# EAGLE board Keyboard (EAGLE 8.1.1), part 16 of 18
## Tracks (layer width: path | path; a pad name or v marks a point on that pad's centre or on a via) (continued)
S$16561 (continued)
  Bottom 0: 240.03,79.83 248.76,71.09
S$16562
  Bottom 0: 248.76,71.09 248.82,71.05
S$16563
  Bottom 0: 248.82,71.05 248.88,71.01
S$16564
  Bottom 0: 248.88,71.01 248.94,70.98
S$16565
  Bottom 0: 248.94,70.98 249.01,70.97
S$16566
  Bottom 0: 249.01,70.97 249.08,70.97
S$16567
  Bottom 0: 249.08,70.97 251.03,70.97
S$16568
  Bottom 0: 251.03,70.97 255.22,66.77
S$16569
  Bottom 0: 255.22,66.77 255.27,66.73
S$16570
  Bottom 0: 255.27,66.73 255.33,66.69
S$16571
  Bottom 0: 255.33,66.69 255.39,66.66
S$16572
  Bottom 0: 255.39,66.66 255.46,66.65
S$16573
  Bottom 0: 255.46,66.65 255.53,66.64
S$16574
  Bottom 0: 255.53,66.64 259.04,66.64
S$16575
  Bottom 0: 259.04,66.64 259.11,66.65
S$16576
  Bottom 0: 259.11,66.65 259.17,66.66
S$16577
  Bottom 0: 259.17,66.66 259.23,66.69
S$16578
  Bottom 0: 259.23,66.69 259.29,66.72
S$16579
  Bottom 0: 259.29,66.72 259.35,66.77
S$16580
  Bottom 0: 259.35,66.77 259.7,67.11
S$16581
  Bottom 0: 259.7,67.11 260.5,67.11
S$16582
  Bottom 0: 260.5,67.11 260.44,67.06
S$16583
  Bottom 0: 260.44,67.06 260.27,66.81
S$16584
  Bottom 0: 260.27,66.81 260.18,66.53
S$16585
  Bottom 0: 260.18,66.53 260.18,66.22
S$16586
  Bottom 0: 260.18,66.22 260.27,65.93
S$16587
  Bottom 0: 260.27,65.93 260.44,65.68
S$16588
  Bottom 0: 260.44,65.68 260.68,65.49
S$16589
  Bottom 0: 260.68,65.49 260.96,65.38
S$16590
  Bottom 0: 260.96,65.38 261.26,65.36
S$16591
  Bottom 0: 261.26,65.36 261.56,65.43
S$16592
  Bottom 0: 261.56,65.43 261.82,65.58
S$16593
  Bottom 0: 261.82,65.58 262.02,65.8
S$16594
  Bottom 0: 262.02,65.8 262.15,66.07
S$16595
  Bottom 0: 262.15,66.07 262.2,66.37
S$16596
  Bottom 0: 262.2,66.37 262.15,66.67
S$16597
  Bottom 0: 262.15,66.67 262.02,66.94
S$16598
  Bottom 0: 262.02,66.94 261.87,67.11
S$16599
  Bottom 0: 261.87,67.11 264.83,67.11
S$16600
  Bottom 0: 264.83,67.11 265.05,66.9
S$16601
  Bottom 0: 265.05,66.9 265.1,66.86
S$16602
  Bottom 0: 265.1,66.86 265.16,66.81
S$16603
  Bottom 0: 265.16,66.81 265.22,66.79
S$16604
  Bottom 0: 265.22,66.79 265.29,66.77
S$16605
  Bottom 0: 265.29,66.77 265.36,66.77
S$16606
  Bottom 0: 265.36,66.77 268.52,66.77
S$16607
  Bottom 0: 268.52,66.77 268.22,66.61
S$16608
  Bottom 0: 268.22,66.61 267.88,66.32
S$16609
  Bottom 0: 267.88,66.32 267.59,65.98
S$16610
  Bottom 0: 267.59,65.98 267.38,65.58
S$16611
  Bottom 0: 267.38,65.58 267.25,65.15
S$16612
  Bottom 0: 267.25,65.15 267.2,64.71
S$16613
  Bottom 0: 267.2,64.71 267.25,64.26
S$16614
  Bottom 0: 267.25,64.26 267.38,63.83
S$16615
  Bottom 0: 267.38,63.83 267.59,63.44
S$16616
  Bottom 0: 267.59,63.44 267.88,63.09
S$16617
  Bottom 0: 267.88,63.09 268.22,62.81
S$16618
  Bottom 0: 268.22,62.81 268.59,62.61
S$16619
  Bottom 0: 268.59,62.61 254.76,62.61
S$16620
  Bottom 0: 254.12,65.36 254.41,65.43
S$16621
  Bottom 0: 254.41,65.43 254.68,65.58
S$16622
  Bottom 0: 254.68,65.58 254.88,65.8
S$16623
  Bottom 0: 254.88,65.8 255.01,66.07
S$16624
  Bottom 0: 255.01,66.07 255.06,66.37
S$16625
  Bottom 0: 255.06,66.37 255.01,66.67
S$16626
  Bottom 0: 255.01,66.67 254.88,66.94
S$16627
  Bottom 0: 254.88,66.94 254.68,67.17
S$16628
  Bottom 0: 254.68,67.17 254.41,67.32
S$16629
  Bottom 0: 254.41,67.32 254.12,67.38
S$16630
  Bottom 0: 254.12,67.38 253.81,67.36
S$16631
  Bottom 0: 253.81,67.36 253.53,67.25
S$16632
  Bottom 0: 253.53,67.25 253.3,67.06
S$16633
  Bottom 0: 253.3,67.06 253.13,66.81
S$16634
  Bottom 0: 253.13,66.81 253.04,66.53
S$16635
  Bottom 0: 253.04,66.53 253.04,66.22
S$16636
  Bottom 0: 253.04,66.22 253.13,65.93
S$16637
  Bottom 0: 253.13,65.93 253.3,65.68
S$16638
  Bottom 0: 253.3,65.68 253.53,65.49
S$16639
  Bottom 0: 253.53,65.49 253.81,65.38
S$16640
  Bottom 0: 253.81,65.38 254.12,65.36
S$16641
  Bottom 0: 255.71,67.53 253.77,69.48
S$16642
  Bottom 0: 253.77,69.48 254.05,69.49
S$16643
  Bottom 0: 254.05,69.49 254.35,69.6
S$16644
  Bottom 0: 254.35,69.6 254.62,69.79
S$16645
  Bottom 0: 254.62,69.79 254.83,70.04
S$16646
  Bottom 0: 254.83,70.04 254.95,70.34
S$16647
  Bottom 0: 254.95,70.34 255,70.66
S$16648
  Bottom 0: 255,70.66 254.95,70.98
S$16649
  Bottom 0: 254.95,70.98 254.83,71.28
S$16650
  Bottom 0: 254.83,71.28 254.62,71.53
S$16651
  Bottom 0: 254.62,71.53 254.35,71.72
S$16652
  Bottom 0: 254.35,71.72 254.05,71.83
S$16653
  Bottom 0: 254.05,71.83 253.72,71.85
S$16654
  Bottom 0: 253.72,71.85 253.47,71.8
S$16655
  Bottom 0: 253.47,71.8 251.83,73.44
S$16656
  Bottom 0: 251.83,73.44 251.76,73.5
S$16657
  Bottom 0: 251.76,73.5 251.69,73.55
S$16658
  Bottom 0: 251.69,73.55 251.6,73.59
S$16659
  Bottom 0: 251.6,73.59 251.52,73.61
S$16660
  Bottom 0: 251.52,73.61 251.42,73.61
S$16661
  Bottom 0: 251.42,73.61 250.56,73.61
S$16662
  Bottom 0: 250.56,73.61 250.53,73.66
S$16663
  Bottom 0: 250.53,73.66 250.33,73.92
S$16664
  Bottom 0: 250.33,73.92 250.07,74.11
S$16665
  Bottom 0: 250.07,74.11 249.76,74.21
S$16666
  Bottom 0: 249.76,74.21 249.44,74.23
S$16667
  Bottom 0: 249.44,74.23 249.12,74.17
S$16668
  Bottom 0: 249.12,74.17 248.83,74.02
S$16669
  Bottom 0: 248.83,74.02 248.59,73.8
S$16670
  Bottom 0: 248.59,73.8 248.42,73.52
S$16671
  Bottom 0: 248.42,73.52 248.33,73.2
S$16672
  Bottom 0: 248.33,73.2 248.33,72.88
S$16673
  Bottom 0: 248.33,72.88 248.37,72.75
S$16674
  Bottom 0: 248.37,72.75 240.91,80.21
S$16675
  Bottom 0: 240.91,80.21 240.98,80.26
S$16676
  Bottom 0: 240.98,80.26 241.19,80.55
S$16677
  Bottom 0: 241.19,80.55 241.32,80.87
S$16678
  Bottom 0: 241.32,80.87 241.36,81.22
S$16679
  Bottom 0: 241.36,81.22 241.32,81.56
S$16680
  Bottom 0: 241.32,81.56 241.19,81.89
S$16681
  Bottom 0: 241.19,81.89 240.98,82.17
S$16682
  Bottom 0: 240.98,82.17 240.71,82.39
S$16683
  Bottom 0: 240.71,82.39 240.4,82.55
S$16684
  Bottom 0: 240.4,82.55 240.05,82.61
S$16685
  Bottom 0: 240.05,82.61 239.74,82.59
S$16686
  Bottom 0: 239.74,82.59 244.05,86.91
S$16687
  Bottom 0: 244.05,86.91 244.29,86.81
S$16688
  Bottom 0: 244.29,86.81 244.59,86.79
S$16689
  Bottom 0: 244.59,86.79 244.89,86.86
S$16690
  Bottom 0: 244.89,86.86 245.15,87.01
S$16691
  Bottom 0: 245.15,87.01 245.36,87.23
S$16692
  Bottom 0: 245.36,87.23 245.49,87.51
S$16693
  Bottom 0: 245.49,87.51 245.53,87.81
S$16694
  Bottom 0: 245.53,87.81 245.49,88.11
S$16695
  Bottom 0: 245.49,88.11 245.36,88.38
S$16696
  Bottom 0: 245.36,88.38 245.19,88.56
S$16697
  Bottom 0: 245.19,88.56 245.59,88.56
S$16698
  Bottom 0: 245.59,88.56 247.1,87.05
S$16699
  Bottom 0: 247.1,87.05 247.17,86.99
S$16700
  Bottom 0: 247.17,86.99 247.25,86.94
S$16701
  Bottom 0: 247.25,86.94 247.33,86.91
S$16702
  Bottom 0: 247.33,86.91 247.41,86.89
S$16703
  Bottom 0: 247.41,86.89 247.5,86.88
S$16704
  Bottom 0: 247.5,86.88 264.62,86.88
S$16705
  Bottom 0: 264.62,86.88 264.71,86.89
S$16706
  Bottom 0: 264.71,86.89 264.79,86.91
S$16707
  Bottom 0: 264.79,86.91 264.87,86.94
S$16708
  Bottom 0: 264.87,86.94 264.95,86.99
S$16709
  Bottom 0: 264.95,86.99 265.01,87.05
S$16710
  Bottom 0: 265.01,87.05 265.71,87.74
S$16711
  Bottom 0: 265.71,87.74 265.84,87.7
S$16712
  Bottom 0: 265.84,87.7 266.13,87.7
S$16713
  Bottom 0: 266.13,87.7 266.05,87.5
S$16714
  Bottom 0: 266.05,87.5 266.05,87.24
S$16715
  Bottom 0: 266.05,87.24 266.14,87.01
S$16716
  Bottom 0: 266.14,87.01 266.32,86.82
S$16717
  Bottom 0: 266.32,86.82 266.54,86.71
S$16718
  Bottom 0: 266.54,86.71 266.75,86.69
S$16719
  Bottom 0: 266.75,86.69 266.75,84.8
S$16720
  Bottom 0: 266.75,84.8 266.63,85.03
S$16721
  Bottom 0: 266.63,85.03 266.34,85.37
S$16722
  Bottom 0: 266.34,85.37 266,85.66
S$16723
  Bottom 0: 266,85.66 265.61,85.87
S$16724
  Bottom 0: 265.61,85.87 265.18,86
S$16725
  Bottom 0: 265.18,86 264.73,86.04
S$16726
  Bottom 0: 264.73,86.04 264.28,86
S$16727
  Bottom 0: 264.28,86 263.86,85.87
S$16728
  Bottom 0: 263.86,85.87 263.46,85.66
S$16729
  Bottom 0: 263.46,85.66 263.12,85.37
S$16730
  Bottom 0: 263.12,85.37 262.83,85.03
S$16731
  Bottom 0: 262.83,85.03 262.62,84.63
S$16732
  Bottom 0: 262.62,84.63 262.49,84.2
S$16733
  Bottom 0: 262.49,84.2 262.44,83.76
S$16734
  Bottom 0: 262.44,83.76 262.49,83.31
S$16735
  Bottom 0: 262.49,83.31 262.62,82.88
S$16736
  Bottom 0: 262.62,82.88 262.83,82.49
S$16737
  Bottom 0: 262.83,82.49 263.12,82.14
S$16738
  Bottom 0: 263.12,82.14 263.46,81.86
S$16739
  Bottom 0: 263.46,81.86 263.86,81.64
S$16740
  Bottom 0: 263.86,81.64 264.28,81.52
S$16741
  Bottom 0: 264.28,81.52 264.73,81.47
S$16742
  Bottom 0: 264.73,81.47 265.18,81.52
S$16743
  Bottom 0: 265.18,81.52 265.48,81.61
S$16744
  Bottom 0: 265.48,81.61 264.38,80.51
S$16745
  Bottom 0: 264.38,80.51 264.33,80.45
S$16746
  Bottom 0: 264.33,80.45 264.3,80.4
S$16747
  Bottom 0: 264.3,80.4 264.27,80.33
S$16748
  Bottom 0: 264.27,80.33 264.25,80.27
S$16749
  Bottom 0: 264.25,80.27 264.25,80.19
S$16750
  Bottom 0: 264.25,80.19 264.25,74.11
S$16751
  Bottom 0: 264.25,74.11 261.89,71.75
S$16752
  Bottom 0: 261.89,71.75 261.67,71.83
S$16753
  Bottom 0: 261.67,71.83 261.34,71.85
S$16754
  Bottom 0: 261.34,71.85 261.02,71.78
S$16755
  Bottom 0: 261.02,71.78 260.73,71.64
S$16756
  Bottom 0: 260.73,71.64 260.5,71.41
S$16757
  Bottom 0: 260.5,71.41 260.33,71.14
S$16758
  Bottom 0: 260.33,71.14 260.24,70.82
S$16759
  Bottom 0: 260.24,70.82 260.24,70.5
S$16760
  Bottom 0: 260.24,70.5 260.33,70.18
S$16761
  Bottom 0: 260.33,70.18 260.5,69.91
S$16762
  Bottom 0: 260.5,69.91 260.73,69.69
S$16763
  Bottom 0: 260.73,69.69 261.02,69.54
S$16764
  Bottom 0: 261.02,69.54 261.34,69.47
S$16765
  Bottom 0: 261.34,69.47 261.67,69.49
S$16766
  Bottom 0: 261.67,69.49 261.97,69.6
S$16767
  Bottom 0: 261.97,69.6 262.24,69.79
S$16768
  Bottom 0: 262.24,69.79 262.44,70.04
S$16769
  Bottom 0: 262.44,70.04 262.57,70.34
S$16770
  Bottom 0: 262.57,70.34 262.62,70.66
S$16771
  Bottom 0: 262.62,70.66 262.57,70.98
S$16772
  Bottom 0: 262.57,70.98 262.51,71.12
S$16773
  Bottom 0: 262.51,71.12 265.01,73.62
S$16774
  Bottom 0: 265.01,73.62 265.05,73.67
S$16775
  Bottom 0: 265.05,73.67 265.09,73.73
S$16776
  Bottom 0: 265.09,73.73 265.11,73.8
S$16777
  Bottom 0: 265.11,73.8 265.13,73.86
S$16778
  Bottom 0: 265.13,73.86 265.13,73.93
S$16779
  Bottom 0: 265.13,73.93 265.13,80.01
S$16780
  Bottom 0: 265.13,80.01 267.5,82.38
S$16781
  Bottom 0: 267.5,82.38 267.55,82.44
S$16782
  Bottom 0: 267.55,82.44 267.59,82.49
S$16783
  Bottom 0: 267.59,82.49 267.61,82.56
S$16784
  Bottom 0: 267.61,82.56 267.63,82.62
S$16785
  Bottom 0: 267.63,82.62 267.64,82.69
S$16786
  Bottom 0: 267.64,82.69 267.64,86.9
S$16787
  Bottom 0: 267.64,86.9 267.63,86.97
S$16788
  Bottom 0: 267.63,86.97 275.62,78.98
S$16789
  Bottom 0: 275.62,78.98 275.62,75.45
S$16790
  Bottom 0: 275.62,75.45 271.05,70.88
S$16791
  Bottom 0: 271.05,70.88 270.92,70.92
S$16792
  Bottom 0: 270.92,70.92 270.6,70.92
S$16793
  Bottom 0: 270.6,70.92 270.29,70.83
S$16794
  Bottom 0: 270.29,70.83 270.01,70.65
S$16795
  Bottom 0: 270.01,70.65 269.8,70.41
S$16796
  Bottom 0: 269.8,70.41 269.69,70.17
S$16797
  Bottom 0: 269.69,70.17 269.49,70.23
S$16798
  Bottom 0: 269.49,70.23 269.36,70.23
S$16799
  Bottom 0: 269.36,70.23 269.36,70.67
S$16800
  Bottom 0: 269.36,70.67 269.35,70.75
S$16801
  Bottom 0: 269.35,70.75 269.31,70.82
S$16802
  Bottom 0: 269.31,70.82 269.26,70.88
S$16803
  Bottom 0: 269.26,70.88 269.19,70.92
S$16804
  Bottom 0: 269.19,70.92 269.11,70.93
S$16805
  Bottom 0: 269.11,70.93 267.4,70.93
S$16806
  Bottom 0: 267.4,70.93 267.4,79.46
S$16807
  Bottom 0: 267.4,79.46 267.92,79.97
S$16808
  Bottom 0: 267.92,79.97 267.95,79.95
S$16809
  Bottom 0: 267.95,79.95 268.28,79.84
S$16810
  Bottom 0: 268.28,79.84 268.62,79.83
S$16811
  Bottom 0: 268.62,79.83 268.97,79.89
S$16812
  Bottom 0: 268.97,79.89 269.29,80.04
S$16813
  Bottom 0: 269.29,80.04 269.56,80.26
S$16814
  Bottom 0: 269.56,80.26 269.77,80.55
S$16815
  Bottom 0: 269.77,80.55 269.89,80.87
S$16816
  Bottom 0: 269.89,80.87 269.94,81.22
S$16817
  Bottom 0: 269.94,81.22 269.89,81.56
S$16818
  Bottom 0: 269.89,81.56 269.77,81.89
S$16819
  Bottom 0: 269.77,81.89 269.56,82.17
S$16820
  Bottom 0: 269.56,82.17 269.29,82.39
S$16821
  Bottom 0: 269.29,82.39 268.97,82.55
S$16822
  Bottom 0: 268.97,82.55 268.62,82.61
S$16823
  Bottom 0: 268.62,82.61 268.28,82.59
S$16824
  Bottom 0: 268.28,82.59 267.95,82.48
S$16825
  Bottom 0: 267.95,82.48 267.65,82.29
S$16826
  Bottom 0: 267.65,82.29 267.41,82.04
S$16827
  Bottom 0: 267.41,82.04 267.24,81.73
S$16828
  Bottom 0: 267.24,81.73 267.15,81.39
S$16829
  Bottom 0: 267.15,81.39 267.15,81.04
S$16830
  Bottom 0: 267.15,81.04 267.24,80.7
S$16831
  Bottom 0: 267.24,80.7 267.29,80.6
S$16832
  Bottom 0: 267.29,80.6 266.65,79.96
S$16833
  Bottom 0: 266.65,79.96 266.61,79.9
S$16834
  Bottom 0: 266.61,79.9 266.57,79.84
S$16835
  Bottom 0: 266.57,79.84 266.54,79.78
S$16836
  Bottom 0: 266.54,79.78 266.52,79.71
S$16837
  Bottom 0: 266.52,79.71 266.52,79.64
S$16838
  Bottom 0: 266.52,79.64 266.52,68.61
S$16839
  Bottom 0: 266.52,68.61 266.52,68.54
S$16840
  Bottom 0: 266.52,68.54 266.54,68.47
S$16841
  Bottom 0: 266.54,68.47 266.57,68.4
S$16842
  Bottom 0: 266.57,68.4 266.61,68.35
S$16843
  Bottom 0: 266.61,68.35 266.65,68.29
S$16844
  Bottom 0: 266.65,68.29 267.29,67.65
S$16845
  Bottom 0: 267.29,67.65 265.55,67.65
S$16846
  Bottom 0: 265.55,67.65 265.33,67.87
S$16847
  Bottom 0: 265.33,67.87 265.27,67.91
S$16848
  Bottom 0: 265.27,67.91 265.21,67.95
S$16849
  Bottom 0: 265.21,67.95 265.15,67.98
S$16850
  Bottom 0: 265.15,67.98 265.09,67.99
S$16851
  Bottom 0: 265.09,67.99 265.01,68
S$16852
  Bottom 0: 265.01,68 259.51,68
S$16853
  Bottom 0: 259.51,68 259.44,67.99
S$16854
  Bottom 0: 259.44,67.99 259.38,67.98
S$16855
  Bottom 0: 259.38,67.98 259.32,67.95
S$16856
  Bottom 0: 259.32,67.95 259.25,67.92
S$16857
  Bottom 0: 259.25,67.92 259.2,67.87
S$16858
  Bottom 0: 259.2,67.87 258.85,67.53
S$16859
  Bottom 0: 258.85,67.53 258.28,67.53
S$16860
  Bottom 0: 258.28,67.53 258.45,67.7
S$16861
  Bottom 0: 258.45,67.7 258.58,67.98
S$16862
  Bottom 0: 258.58,67.98 258.62,68.28
S$16863
  Bottom 0: 258.62,68.28 258.58,68.58
S$16864
  Bottom 0: 258.58,68.58 258.45,68.85
S$16865
  Bottom 0: 258.45,68.85 258.24,69.07
S$16866
  Bottom 0: 258.24,69.07 258.05,69.18
S$16867
  Bottom 0: 258.05,69.18 258.05,73.91
S$16868
  Bottom 0: 258.05,73.91 261.57,77.43
S$16869
  Bottom 0: 261.57,77.43 261.6,77.41
S$16870
  Bottom 0: 261.6,77.41 261.93,77.31
S$16871
  Bottom 0: 261.93,77.31 262.27,77.28
S$16872
  Bottom 0: 262.27,77.28 262.62,77.35
S$16873
  Bottom 0: 262.62,77.35 262.94,77.5
S$16874
  Bottom 0: 262.94,77.5 263.21,77.72
S$16875
  Bottom 0: 263.21,77.72 263.42,78.01
S$16876
  Bottom 0: 263.42,78.01 263.54,78.33
S$16877
  Bottom 0: 263.54,78.33 263.59,78.68
S$16878
  Bottom 0: 263.59,78.68 263.54,79.02
S$16879
  Bottom 0: 263.54,79.02 263.42,79.35
S$16880
  Bottom 0: 263.42,79.35 263.21,79.63
S$16881
  Bottom 0: 263.21,79.63 262.94,79.86
S$16882
  Bottom 0: 262.94,79.86 262.62,80.01
S$16883
  Bottom 0: 262.62,80.01 262.27,80.07
S$16884
  Bottom 0: 262.27,80.07 261.93,80.05
S$16885
  Bottom 0: 261.93,80.05 261.6,79.94
S$16886
  Bottom 0: 261.6,79.94 261.3,79.75
S$16887
  Bottom 0: 261.3,79.75 261.06,79.5
S$16888
  Bottom 0: 261.06,79.5 260.89,79.19
S$16889
  Bottom 0: 260.89,79.19 260.81,78.85
S$16890
  Bottom 0: 260.81,78.85 260.81,78.5
S$16891
  Bottom 0: 260.81,78.5 260.89,78.16
S$16892
  Bottom 0: 260.89,78.16 260.94,78.06
S$16893
  Bottom 0: 260.94,78.06 257.29,74.41
S$16894
  Bottom 0: 257.29,74.41 257.25,74.35
S$16895
  Bottom 0: 257.25,74.35 257.21,74.29
S$16896
  Bottom 0: 257.21,74.29 257.19,74.23
S$16897
  Bottom 0: 257.19,74.23 257.17,74.17
S$16898
  Bottom 0: 257.17,74.17 257.17,74.09
S$16899
  Bottom 0: 257.17,74.09 257.17,69.18
S$16900
  Bottom 0: 257.17,69.18 257.1,69.16
S$16901
  Bottom 0: 257.1,69.16 256.86,68.97
S$16902
  Bottom 0: 256.86,68.97 256.69,68.72
S$16903
  Bottom 0: 256.69,68.72 256.6,68.43
S$16904
  Bottom 0: 256.6,68.43 256.6,68.12
S$16905
  Bottom 0: 256.6,68.12 256.69,67.83
S$16906
  Bottom 0: 256.69,67.83 256.86,67.59
S$16907
  Bottom 0: 256.86,67.59 256.94,67.53
S$16908
  Bottom 0: 256.94,67.53 255.71,67.53
S$16909
  Bottom 0: 244.59,79.17 244.89,79.24
S$16910
  Bottom 0: 244.89,79.24 245.15,79.39
S$16911
  Bottom 0: 245.15,79.39 245.36,79.61
S$16912
  Bottom 0: 245.36,79.61 245.49,79.89
S$16913
  Bottom 0: 245.49,79.89 245.53,80.19
S$16914
  Bottom 0: 245.53,80.19 245.49,80.48
S$16915
  Bottom 0: 245.49,80.48 245.36,80.76
S$16916
  Bottom 0: 245.36,80.76 245.15,80.98
S$16917
  Bottom 0: 245.15,80.98 244.89,81.13
S$16918
  Bottom 0: 244.89,81.13 244.59,81.2
S$16919
  Bottom 0: 244.59,81.2 244.29,81.18
S$16920
  Bottom 0: 244.29,81.18 244.01,81.06
S$16921
  Bottom 0: 244.01,81.06 243.77,80.88
S$16922
  Bottom 0: 243.77,80.88 243.6,80.63
S$16923
  Bottom 0: 243.6,80.63 243.51,80.34
S$16924
  Bottom 0: 243.51,80.34 243.51,80.03
S$16925
  Bottom 0: 243.51,80.03 243.6,79.74
S$16926
  Bottom 0: 243.6,79.74 243.77,79.49
S$16927
  Bottom 0: 243.77,79.49 244.01,79.31
S$16928
  Bottom 0: 244.01,79.31 244.29,79.19
S$16929
  Bottom 0: 244.29,79.19 244.59,79.17
S$16930
  Bottom 0: 207.45,68.93 207.45,70.67
S$16931
  Bottom 0: 207.45,70.67 207.44,70.75
S$16932
  Bottom 0: 207.44,70.75 207.4,70.82
S$16933
  Bottom 0: 207.4,70.82 207.35,70.88
S$16934
  Bottom 0: 207.35,70.88 207.28,70.92
S$16935
  Bottom 0: 207.28,70.92 207.2,70.93
S$16936
  Bottom 0: 207.2,70.93 206.75,70.93
S$16937
  Bottom 0: 206.75,70.93 206.75,71.06
S$16938
  Bottom 0: 206.75,71.06 206.69,71.28
S$16939
  Bottom 0: 206.69,71.28 206.53,71.44
S$16940
  Bottom 0: 206.53,71.44 206.31,71.5
S$16941
  Bottom 0: 206.31,71.5 205.97,71.5
S$16942
  Bottom 0: 205.97,71.5 204.88,72.59
S$16943
  Bottom 0: 204.88,72.59 204.94,72.72
S$16944
  Bottom 0: 204.94,72.72 204.99,73.04
S$16945
  Bottom 0: 204.99,73.04 204.94,73.36
S$16946
  Bottom 0: 204.94,73.36 204.81,73.66
S$16947
  Bottom 0: 204.81,73.66 204.6,73.92
S$16948
  Bottom 0: 204.6,73.92 204.34,74.11
S$16949
  Bottom 0: 204.34,74.11 204.04,74.21
S$16950
  Bottom 0: 204.04,74.21 203.71,74.23
S$16951
  Bottom 0: 203.71,74.23 203.39,74.17
S$16952
  Bottom 0: 203.39,74.17 203.1,74.02
S$16953
  Bottom 0: 203.1,74.02 202.87,73.8
S$16954
  Bottom 0: 202.87,73.8 202.69,73.52
S$16955
  Bottom 0: 202.69,73.52 202.61,73.2
S$16956
  Bottom 0: 202.61,73.2 202.61,72.88
S$16957
  Bottom 0: 202.61,72.88 202.69,72.56
S$16958
  Bottom 0: 202.69,72.56 202.87,72.29
S$16959
  Bottom 0: 202.87,72.29 203.1,72.07
S$16960
  Bottom 0: 203.1,72.07 203.39,71.92
S$16961
  Bottom 0: 203.39,71.92 203.71,71.85
S$16962
  Bottom 0: 203.71,71.85 204.04,71.87
S$16963
  Bottom 0: 204.04,71.87 204.25,71.95
S$16964
  Bottom 0: 204.25,71.95 205.31,70.9
S$16965
  Bottom 0: 205.31,70.9 205.28,70.88
S$16966
  Bottom 0: 205.28,70.88 205.22,70.82
S$16967
  Bottom 0: 205.22,70.82 205.18,70.75
S$16968
  Bottom 0: 205.18,70.75 205.17,70.67
S$16969
  Bottom 0: 205.17,70.67 205.17,69.18
S$16970
  Bottom 0: 205.17,69.18 198.67,75.68
S$16971
  Bottom 0: 198.67,75.68 198.67,78.82
S$16972
  Bottom 0: 198.67,78.82 198.67,78.89
S$16973
  Bottom 0: 198.67,78.89 198.65,78.96
S$16974
  Bottom 0: 198.65,78.96 198.62,79.02
S$16975
  Bottom 0: 198.62,79.02 198.59,79.08
S$16976
  Bottom 0: 198.59,79.08 198.54,79.13
S$16977
  Bottom 0: 198.54,79.13 196.02,81.65
S$16978
  Bottom 0: 196.02,81.65 196.02,82.73
S$16979
  Bottom 0: 196.02,82.73 196.16,82.49
S$16980
  Bottom 0: 196.16,82.49 196.44,82.14
S$16981
  Bottom 0: 196.44,82.14 196.79,81.86
S$16982
  Bottom 0: 196.79,81.86 197.18,81.64
S$16983
  Bottom 0: 197.18,81.64 197.61,81.52
S$16984
  Bottom 0: 197.61,81.52 198.06,81.47
S$16985
  Bottom 0: 198.06,81.47 198.5,81.52
S$16986
  Bottom 0: 198.5,81.52 198.93,81.64
S$16987
  Bottom 0: 198.93,81.64 199.33,81.86
S$16988
  Bottom 0: 199.33,81.86 199.6,82.08
S$16989
  Bottom 0: 199.6,82.08 199.6,80.48
S$16990
  Bottom 0: 199.6,80.48 199.6,80.39
S$16991
  Bottom 0: 199.6,80.39 199.63,80.31
S$16992
  Bottom 0: 199.63,80.31 199.66,80.23
S$16993
  Bottom 0: 199.66,80.23 199.71,80.15
S$16994
  Bottom 0: 199.71,80.15 199.77,80.08
S$16995
  Bottom 0: 199.77,80.08 208.28,71.58
S$16996
  Bottom 0: 208.28,71.58 208.28,70.77
S$16997
  Bottom 0: 208.28,70.77 208.1,70.65
S$16998
  Bottom 0: 208.1,70.65 207.89,70.41
S$16999
  Bottom 0: 207.89,70.41 207.75,70.11
S$17000
  Bottom 0: 207.75,70.11 207.71,69.79
S$17001
  Bottom 0: 207.71,69.79 207.75,69.47
S$17002
  Bottom 0: 207.75,69.47 207.89,69.16
S$17003
  Bottom 0: 207.89,69.16 208.09,68.93
S$17004
  Bottom 0: 208.09,68.93 207.45,68.93
S$17005
  Bottom 0: 201.81,74.23 202.13,74.24
S$17006
  Bottom 0: 202.13,74.24 202.44,74.35
S$17007
  Bottom 0: 202.44,74.35 202.7,74.54
S$17008
  Bottom 0: 202.7,74.54 202.91,74.8
S$17009
  Bottom 0: 202.91,74.8 203.03,75.09
S$17010
  Bottom 0: 203.03,75.09 203.08,75.42
S$17011
  Bottom 0: 203.08,75.42 203.03,75.73
S$17012
  Bottom 0: 203.03,75.73 202.91,76.03
S$17013
  Bottom 0: 202.91,76.03 202.7,76.29
S$17014
  Bottom 0: 202.7,76.29 202.44,76.48
S$17015
  Bottom 0: 202.44,76.48 202.13,76.58
S$17016
  Bottom 0: 202.13,76.58 201.81,76.6
S$17017
  Bottom 0: 201.81,76.6 201.49,76.54
S$17018
  Bottom 0: 201.49,76.54 201.19,76.39
S$17019
  Bottom 0: 201.19,76.39 200.96,76.17
S$17020
  Bottom 0: 200.96,76.17 200.79,75.89
S$17021
  Bottom 0: 200.79,75.89 200.7,75.58
S$17022
  Bottom 0: 200.7,75.58 200.7,75.25
S$17023
  Bottom 0: 200.7,75.25 200.79,74.94
S$17024
  Bottom 0: 200.79,74.94 200.96,74.66
S$17025
  Bottom 0: 200.96,74.66 201.19,74.44
S$17026
  Bottom 0: 201.19,74.44 201.49,74.29
S$17027
  Bottom 0: 201.49,74.29 201.81,74.23
S$17028
  Bottom 0: 150.3,69.19 150.3,70.67
S$17029
  Bottom 0: 150.3,70.67 150.29,70.75
S$17030
  Bottom 0: 150.29,70.75 150.25,70.82
S$17031
  Bottom 0: 150.25,70.82 150.2,70.88
S$17032
  Bottom 0: 150.2,70.88 150.12,70.92
S$17033
  Bottom 0: 150.12,70.92 150.05,70.93
S$17034
  Bottom 0: 150.05,70.93 149.6,70.93
S$17035
  Bottom 0: 149.6,70.93 149.6,71.06
S$17036
  Bottom 0: 149.6,71.06 149.54,71.28
S$17037
  Bottom 0: 149.54,71.28 149.38,71.44
S$17038
  Bottom 0: 149.38,71.44 149.16,71.5
S$17039
  Bottom 0: 149.16,71.5 148.81,71.5
S$17040
  Bottom 0: 148.81,71.5 147.72,72.59
S$17041
  Bottom 0: 147.72,72.59 147.78,72.72
S$17042
  Bottom 0: 147.78,72.72 147.83,73.04
S$17043
  Bottom 0: 147.83,73.04 147.78,73.36
S$17044
  Bottom 0: 147.78,73.36 147.66,73.66
S$17045
  Bottom 0: 147.66,73.66 147.45,73.92
S$17046
  Bottom 0: 147.45,73.92 147.41,73.95
S$17047
  Bottom 0: 147.41,73.95 149.14,73.95
S$17048
  Bottom 0: 149.14,73.95 152.4,70.68
S$17049
  Bottom 0: 152.4,70.68 152.17,70.83
S$17050
  Bottom 0: 152.17,70.83 151.86,70.92
S$17051
  Bottom 0: 151.86,70.92 151.54,70.92
S$17052
  Bottom 0: 151.54,70.92 151.23,70.83
S$17053
  Bottom 0: 151.23,70.83 150.95,70.65
S$17054
  Bottom 0: 150.95,70.65 150.74,70.41
S$17055
  Bottom 0: 150.74,70.41 150.6,70.11
S$17056
  Bottom 0: 150.6,70.11 150.56,69.79
S$17057
  Bottom 0: 150.56,69.79 150.6,69.48
S$17058
  Bottom 0: 150.6,69.48 150.3,69.19
S$17059
  Bottom 0: 316.85,70.43 316.85,70.66
S$17060
  Bottom 0: 316.85,70.66 316.84,70.74
S$17061
  Bottom 0: 316.84,70.74 316.8,70.81
S$17062
  Bottom 0: 316.8,70.81 316.74,70.86
S$17063
  Bottom 0: 316.74,70.86 316.67,70.9
S$17064
  Bottom 0: 316.67,70.9 316.59,70.91
S$17065
  Bottom 0: 316.59,70.91 315.52,70.91
S$17066
  Bottom 0: 315.52,70.91 315.52,71.04
S$17067
  Bottom 0: 315.52,71.04 315.5,71.1
S$17068
  Bottom 0: 315.5,71.1 315.5,71.16
S$17069
  Bottom 0: 315.5,71.16 315.47,71.21
S$17070
  Bottom 0: 315.47,71.21 315.45,71.26
S$17071
  Bottom 0: 315.45,71.26 315.43,71.3
S$17072
  Bottom 0: 315.43,71.3 315.39,71.36
S$17073
  Bottom 0: 315.39,71.36 314.34,72.4
S$17074
  Bottom 0: 314.34,72.4 314.36,72.42
S$17075
  Bottom 0: 314.36,72.42 314.49,72.72
S$17076
  Bottom 0: 314.49,72.72 314.54,73.04
S$17077
  Bottom 0: 314.54,73.04 314.49,73.36
S$17078
  Bottom 0: 314.49,73.36 314.36,73.66
S$17079
  Bottom 0: 314.36,73.66 314.15,73.92
S$17080
  Bottom 0: 314.15,73.92 313.89,74.11
S$17081
  Bottom 0: 313.89,74.11 313.58,74.21
S$17082
  Bottom 0: 313.58,74.21 313.3,74.23
S$17083
  Bottom 0: 313.3,74.23 313.58,74.24
S$17084
  Bottom 0: 313.58,74.24 313.89,74.35
S$17085
  Bottom 0: 313.89,74.35 314.15,74.54
S$17086
  Bottom 0: 314.15,74.54 314.36,74.8
S$17087
  Bottom 0: 314.36,74.8 314.49,75.09
S$17088
  Bottom 0: 314.49,75.09 314.54,75.42
S$17089
  Bottom 0: 314.54,75.42 314.49,75.73
S$17090
  Bottom 0: 314.49,75.73 314.36,76.03
S$17091
  Bottom 0: 314.36,76.03 314.15,76.29
S$17092
  Bottom 0: 314.15,76.29 313.89,76.48
S$17093
  Bottom 0: 313.89,76.48 313.58,76.58
S$17094
  Bottom 0: 313.58,76.58 313.26,76.6
S$17095
  Bottom 0: 313.26,76.6 312.94,76.54
S$17096
  Bottom 0: 312.94,76.54 312.88,76.51
S$17097
  Bottom 0: 312.88,76.51 312.73,76.66
S$17098
  Bottom 0: 312.73,76.66 312.73,77.78
S$17099
  Bottom 0: 312.73,77.78 312.92,77.58
S$17100
  Bottom 0: 312.92,77.58 313.21,77.4
S$17101
  Bottom 0: 313.21,77.4 313.54,77.29
S$17102
  Bottom 0: 313.54,77.29 313.89,77.27
S$17103
  Bottom 0: 313.89,77.27 314.19,77.33
S$17104
  Bottom 0: 314.19,77.33 314.3,77.29
S$17105
  Bottom 0: 314.3,77.29 314.65,77.27
S$17106
  Bottom 0: 314.65,77.27 315,77.33
S$17107
  Bottom 0: 315,77.33 315.31,77.48
S$17108
  Bottom 0: 315.31,77.48 315.58,77.71
S$17109
  Bottom 0: 315.58,77.71 315.79,77.99
S$17110
  Bottom 0: 315.79,77.99 315.92,78.32
S$17111
  Bottom 0: 315.92,78.32 315.96,78.66
S$17112
  Bottom 0: 315.96,78.66 315.92,79.01
S$17113
  Bottom 0: 315.92,79.01 315.79,79.33
S$17114
  Bottom 0: 315.79,79.33 315.58,79.62
S$17115
  Bottom 0: 315.58,79.62 315.31,79.84
S$17116
  Bottom 0: 315.31,79.84 315,79.99
S$17117
  Bottom 0: 315,79.99 314.65,80.05
S$17118
  Bottom 0: 314.65,80.05 314.3,80.03
S$17119
  Bottom 0: 314.3,80.03 314.19,80
S$17120
  Bottom 0: 314.19,80 313.89,80.05
S$17121
  Bottom 0: 313.89,80.05 313.54,80.03
S$17122
  Bottom 0: 313.54,80.03 313.21,79.93
S$17123
  Bottom 0: 313.21,79.93 312.92,79.74
S$17124
  Bottom 0: 312.92,79.74 312.73,79.54
S$17125
  Bottom 0: 312.73,79.54 312.73,84.58
S$17126
  Bottom 0: 312.73,84.58 314.47,86.32
S$17127
  Bottom 0: 314.47,86.32 313.32,85.17
S$17128
  Bottom 0: 313.32,85.17 313.26,85.1
S$17129
  Bottom 0: 313.26,85.1 313.21,85.03
S$17130
  Bottom 0: 313.21,85.03 313.17,84.94
S$17131
  Bottom 0: 313.17,84.94 313.15,84.85
S$17132
  Bottom 0: 313.15,84.85 313.15,84.77
S$17133
  Bottom 0: 313.15,84.77 313.15,82.75
S$17134
  Bottom 0: 313.15,82.75 313.15,82.65
S$17135
  Bottom 0: 313.15,82.65 313.17,82.57
S$17136
  Bottom 0: 313.17,82.57 313.21,82.49
S$17137
  Bottom 0: 313.21,82.49 313.26,82.41
S$17138
  Bottom 0: 313.26,82.41 313.32,82.34
S$17139
  Bottom 0: 313.32,82.34 317.81,77.85
S$17140
  Bottom 0: 317.81,77.85 317.81,70.75
S$17141
  Bottom 0: 317.81,70.75 317.69,70.78
S$17142
  Bottom 0: 317.69,70.78 317.39,70.76
S$17143
  Bottom 0: 317.39,70.76 317.11,70.65
S$17144
  Bottom 0: 317.11,70.65 316.87,70.46
S$17145
  Bottom 0: 316.87,70.46 316.85,70.43
S$17146
  Bottom 0: 319.21,70.54 319.12,70.64
S$17147
  Bottom 0: 319.12,70.64 318.94,70.75
S$17148
  Bottom 0: 318.94,70.75 318.94,78.09
S$17149
  Bottom 0: 318.94,78.09 318.94,78.18
S$17150
  Bottom 0: 318.94,78.18 318.92,78.27
S$17151
  Bottom 0: 318.92,78.27 318.88,78.35
S$17152
  Bottom 0: 318.88,78.35 318.84,78.42
S$17153
  Bottom 0: 318.84,78.42 318.78,78.49
S$17154
  Bottom 0: 318.78,78.49 315.71,81.56
S$17155
  Bottom 0: 315.71,81.56 315.89,81.5
S$17156
  Bottom 0: 315.89,81.5 316.34,81.45
S$17157
  Bottom 0: 316.34,81.45 316.72,81.5
S$17158
  Bottom 0: 316.72,81.5 317.1,81.45
S$17159
  Bottom 0: 317.1,81.45 317.55,81.5
S$17160
  Bottom 0: 317.55,81.5 317.97,81.63
S$17161
  Bottom 0: 317.97,81.63 318.37,81.84
S$17162
  Bottom 0: 318.37,81.84 318.72,82.13
S$17163
  Bottom 0: 318.72,82.13 319,82.47
S$17164
  Bottom 0: 319,82.47 319.21,82.87
S$17165
  Bottom 0: 319.21,82.87 319.34,83.29
S$17166
  Bottom 0: 319.34,83.29 319.39,83.74
S$17167
  Bottom 0: 319.39,83.74 319.34,84.19
S$17168
  Bottom 0: 319.34,84.19 319.3,84.34
S$17169
  Bottom 0: 319.3,84.34 321.05,82.59
S$17170
  Bottom 0: 321.05,82.59 321,82.59
S$17171
  Bottom 0: 321,82.59 320.65,82.57
S$17172
  Bottom 0: 320.65,82.57 320.55,82.54
S$17173
  Bottom 0: 320.55,82.54 320.24,82.59
S$17174
  Bottom 0: 320.24,82.59 319.89,82.57
S$17175
  Bottom 0: 319.89,82.57 319.56,82.47
S$17176
  Bottom 0: 319.56,82.47 319.26,82.28
S$17177
  Bottom 0: 319.26,82.28 319.03,82.02
S$17178
  Bottom 0: 319.03,82.02 318.85,81.71
S$17179
  Bottom 0: 318.85,81.71 318.77,81.37
S$17180
  Bottom 0: 318.77,81.37 318.77,81.03
S$17181
  Bottom 0: 318.77,81.03 318.85,80.69
S$17182
  Bottom 0: 318.85,80.69 319.03,80.38
S$17183
  Bottom 0: 319.03,80.38 319.21,80.19
S$17184
  Bottom 0: 319.21,80.19 319.21,70.54
S$17185
  Bottom 0: 194.9,73.16 193.67,74.39
S$17186
  Bottom 0: 193.67,74.39 193.87,74.29
S$17187
  Bottom 0: 193.87,74.29 194.19,74.23
S$17188
  Bottom 0: 194.19,74.23 194.51,74.24
S$17189
  Bottom 0: 194.51,74.24 194.81,74.35
S$17190
  Bottom 0: 194.81,74.35 195.08,74.54
S$17191
  Bottom 0: 195.08,74.54 195.28,74.8
S$17192
  Bottom 0: 195.28,74.8 195.41,75.09
S$17193
  Bottom 0: 195.41,75.09 195.46,75.42
S$17194
  Bottom 0: 195.46,75.42 195.41,75.73
S$17195
  Bottom 0: 195.41,75.73 195.28,76.03
S$17196
  Bottom 0: 195.28,76.03 195.08,76.29
S$17197
  Bottom 0: 195.08,76.29 194.81,76.48
S$17198
  Bottom 0: 194.81,76.48 194.51,76.58
S$17199
  Bottom 0: 194.51,76.58 194.31,76.59
S$17200
  Bottom 0: 194.31,76.59 194.31,77.99
S$17201
  Bottom 0: 194.31,77.99 194.39,77.85
S$17202
  Bottom 0: 194.39,77.85 194.63,77.6
S$17203
  Bottom 0: 194.63,77.6 194.92,77.41
S$17204
  Bottom 0: 194.92,77.41 195.25,77.31
S$17205
  Bottom 0: 195.25,77.31 195.6,77.28
S$17206
  Bottom 0: 195.6,77.28 195.95,77.35
S$17207
  Bottom 0: 195.95,77.35 196.26,77.5
S$17208
  Bottom 0: 196.26,77.5 196.53,77.72
S$17209
  Bottom 0: 196.53,77.72 196.74,78.01
S$17210
  Bottom 0: 196.74,78.01 196.87,78.33
S$17211
  Bottom 0: 196.87,78.33 196.91,78.68
S$17212
  Bottom 0: 196.91,78.68 196.87,79.02
S$17213
  Bottom 0: 196.87,79.02 196.74,79.35
S$17214
  Bottom 0: 196.74,79.35 196.53,79.63
S$17215
  Bottom 0: 196.53,79.63 196.26,79.86
S$17216
  Bottom 0: 196.26,79.86 195.95,80.01
S$17217
  Bottom 0: 195.95,80.01 195.6,80.07
S$17218
  Bottom 0: 195.6,80.07 195.25,80.05
S$17219
  Bottom 0: 195.25,80.05 194.92,79.94
S$17220
  Bottom 0: 194.92,79.94 194.63,79.75
S$17221
  Bottom 0: 194.63,79.75 194.39,79.5
S$17222
  Bottom 0: 194.39,79.5 194.31,79.36
S$17223
  Bottom 0: 194.31,79.36 194.31,84.47
S$17224
  Bottom 0: 194.31,84.47 197.1,87.25
S$17225
  Bottom 0: 197.1,87.25 197.13,87.31
S$17226
  Bottom 0: 197.13,87.31 197.17,87.35
S$17227
  Bottom 0: 197.17,87.35 197.18,87.39
S$17228
  Bottom 0: 197.18,87.39 197.21,87.45
S$17229
  Bottom 0: 197.21,87.45 197.21,87.51
S$17230
  Bottom 0: 197.21,87.51 197.23,87.57
S$17231
  Bottom 0: 197.23,87.57 197.23,87.69
S$17232
  Bottom 0: 197.23,87.69 197.6,87.69
S$17233
  Bottom 0: 197.6,87.69 197.6,87.33
S$17234
  Bottom 0: 197.6,87.33 195.27,85
S$17235
  Bottom 0: 195.27,85 195.22,84.94
S$17236
  Bottom 0: 195.22,84.94 195.19,84.88
S$17237
  Bottom 0: 195.19,84.88 195.16,84.82
S$17238
  Bottom 0: 195.16,84.82 195.15,84.75
S$17239
  Bottom 0: 195.15,84.75 195.14,84.68
S$17240
  Bottom 0: 195.14,84.68 195.14,81.47
S$17241
  Bottom 0: 195.14,81.47 195.15,81.39
S$17242
  Bottom 0: 195.15,81.39 195.16,81.33
S$17243
  Bottom 0: 195.16,81.33 195.19,81.27
S$17244
  Bottom 0: 195.19,81.27 195.22,81.21
S$17245
  Bottom 0: 195.22,81.21 195.27,81.15
S$17246
  Bottom 0: 195.27,81.15 197.79,78.63
S$17247
  Bottom 0: 197.79,78.63 197.79,75.5
S$17248
  Bottom 0: 197.79,75.5 197.79,75.43
S$17249
  Bottom 0: 197.79,75.43 197.81,75.36
S$17250
  Bottom 0: 197.81,75.36 197.83,75.3
S$17251
  Bottom 0: 197.83,75.3 197.87,75.24
S$17252
  Bottom 0: 197.87,75.24 197.91,75.19
S$17253
  Bottom 0: 197.91,75.19 199.94,73.16
S$17254
  Bottom 0: 199.94,73.16 194.9,73.16
S$17255
  Bottom 0: 79.09,73.61 79.06,73.66
S$17256
  Bottom 0: 79.06,73.66 78.86,73.92
S$17257
  Bottom 0: 78.86,73.92 78.59,74.11
S$17258
  Bottom 0: 78.59,74.11 78.29,74.21
S$17259
  Bottom 0: 78.29,74.21 77.97,74.23
S$17260
  Bottom 0: 77.97,74.23 77.71,74.18
S$17261
  Bottom 0: 77.71,74.18 75.7,76.19
S$17262
  Bottom 0: 75.7,76.19 75.64,76.25
S$17263
  Bottom 0: 75.64,76.25 75.56,76.29
S$17264
  Bottom 0: 75.56,76.29 75.48,76.33
S$17265
  Bottom 0: 75.48,76.33 75.39,76.35
S$17266
  Bottom 0: 75.39,76.35 75.3,76.36
S$17267
  Bottom 0: 75.3,76.36 69.25,76.36
S$17268
  Bottom 0: 69.25,76.36 69.07,76.48
S$17269
  Bottom 0: 69.07,76.48 68.77,76.59
S$17270
  Bottom 0: 68.77,76.59 68.44,76.61
S$17271
  Bottom 0: 68.44,76.61 68.12,76.54
S$17272
  Bottom 0: 68.12,76.54 68.11,76.53
S$17273
  Bottom 0: 68.11,76.53 81.22,89.65
S$17274
  Bottom 0: 81.22,89.65 81.35,89.65
S$17275
  Bottom 0: 81.35,89.65 81.35,87.95
S$17276
  Bottom 0: 81.35,87.95 81.36,87.87
S$17277
  Bottom 0: 81.36,87.87 81.4,87.8
S$17278
  Bottom 0: 81.4,87.8 81.45,87.74
S$17279
  Bottom 0: 81.45,87.74 81.53,87.7
S$17280
  Bottom 0: 81.53,87.7 81.6,87.69
S$17281
  Bottom 0: 81.6,87.69 81.99,87.69
S$17282
  Bottom 0: 81.99,87.69 79.32,85.03
S$17283
  Bottom 0: 79.32,85.03 79.28,84.98
S$17284
  Bottom 0: 79.28,84.98 79.25,84.92
S$17285
  Bottom 0: 79.25,84.92 79.22,84.85
S$17286
  Bottom 0: 79.22,84.85 79.2,84.79
S$17287
  Bottom 0: 79.2,84.79 79.2,84.72
S$17288
  Bottom 0: 79.2,84.72 79.2,76.33
S$17289
  Bottom 0: 79.2,76.33 79.03,76.17
S$17290
  Bottom 0: 79.03,76.17 78.86,75.89
S$17291
  Bottom 0: 78.86,75.89 78.77,75.58
S$17292
  Bottom 0: 78.77,75.58 78.77,75.26
S$17293
  Bottom 0: 78.77,75.26 78.86,74.94
S$17294
  Bottom 0: 78.86,74.94 79.03,74.67
S$17295
  Bottom 0: 79.03,74.67 79.27,74.44
S$17296
  Bottom 0: 79.27,74.44 79.56,74.3
S$17297
  Bottom 0: 79.56,74.3 79.88,74.23
S$17298
  Bottom 0: 79.88,74.23 80.2,74.25
S$17299
  Bottom 0: 80.2,74.25 80.5,74.36
S$17300
  Bottom 0: 80.5,74.36 80.77,74.55
S$17301
  Bottom 0: 80.77,74.55 80.97,74.8
S$17302
  Bottom 0: 80.97,74.8 81.1,75.1
S$17303
  Bottom 0: 81.1,75.1 81.15,75.42
S$17304
  Bottom 0: 81.15,75.42 81.1,75.74
S$17305
  Bottom 0: 81.1,75.74 80.97,76.04
S$17306
  Bottom 0: 80.97,76.04 80.77,76.29
S$17307
  Bottom 0: 80.77,76.29 80.5,76.48
S$17308
  Bottom 0: 80.5,76.48 80.2,76.59
S$17309
  Bottom 0: 80.2,76.59 80.08,76.59
S$17310
  Bottom 0: 80.08,76.59 80.08,77.87
S$17311
  Bottom 0: 80.08,77.87 80.09,77.85
S$17312
  Bottom 0: 80.09,77.85 80.33,77.6
S$17313
  Bottom 0: 80.33,77.6 80.62,77.41
S$17314
  Bottom 0: 80.62,77.41 80.96,77.31
S$17315
  Bottom 0: 80.96,77.31 81.31,77.28
S$17316
  Bottom 0: 81.31,77.28 81.65,77.35
S$17317
  Bottom 0: 81.65,77.35 81.97,77.5
S$17318
  Bottom 0: 81.97,77.5 82.24,77.72
S$17319
  Bottom 0: 82.24,77.72 82.45,78.01
S$17320
  Bottom 0: 82.45,78.01 82.57,78.33
S$17321
  Bottom 0: 82.57,78.33 82.62,78.68
S$17322
  Bottom 0: 82.62,78.68 82.57,79.02
S$17323
  Bottom 0: 82.57,79.02 82.45,79.35
S$17324
  Bottom 0: 82.45,79.35 82.24,79.63
S$17325
  Bottom 0: 82.24,79.63 81.97,79.86
S$17326
  Bottom 0: 81.97,79.86 81.65,80.01
S$17327
  Bottom 0: 81.65,80.01 81.31,80.07
S$17328
  Bottom 0: 81.31,80.07 80.96,80.05
S$17329
  Bottom 0: 80.96,80.05 80.62,79.94
S$17330
  Bottom 0: 80.62,79.94 80.33,79.75
S$17331
  Bottom 0: 80.33,79.75 80.09,79.5
S$17332
  Bottom 0: 80.09,79.5 80.08,79.48
S$17333
  Bottom 0: 80.08,79.48 80.08,84.53
S$17334
  Bottom 0: 80.08,84.53 82.81,87.25
S$17335
  Bottom 0: 82.81,87.25 82.84,87.32
S$17336
  Bottom 0: 82.84,87.32 82.87,87.35
S$17337
  Bottom 0: 82.87,87.35 82.88,87.39
S$17338
  Bottom 0: 82.88,87.39 82.92,87.45
S$17339
  Bottom 0: 82.92,87.45 82.92,87.51
S$17340
  Bottom 0: 82.92,87.51 82.93,87.57
S$17341
  Bottom 0: 82.93,87.57 82.93,87.69
S$17342
  Bottom 0: 82.93,87.69 83.38,87.69
S$17343
  Bottom 0: 83.38,87.69 83.46,87.7
S$17344
  Bottom 0: 83.46,87.7 83.53,87.74
S$17345
  Bottom 0: 83.53,87.74 83.58,87.8
S$17346
  Bottom 0: 83.58,87.8 83.62,87.87
S$17347
  Bottom 0: 83.62,87.87 83.64,87.95
S$17348
  Bottom 0: 83.64,87.95 83.64,89.65
S$17349
  Bottom 0: 83.64,89.65 84.24,89.65
S$17350
  Bottom 0: 84.24,89.65 84.07,89.46
S$17351
  Bottom 0: 84.07,89.46 83.93,89.16
S$17352
  Bottom 0: 83.93,89.16 83.89,88.84
S$17353
  Bottom 0: 83.89,88.84 83.93,88.52
S$17354
  Bottom 0: 83.93,88.52 84.07,88.22
S$17355
  Bottom 0: 84.07,88.22 84.28,87.97
S$17356
  Bottom 0: 84.28,87.97 84.56,87.8
S$17357
  Bottom 0: 84.56,87.8 84.87,87.7
S$17358
  Bottom 0: 84.87,87.7 85.19,87.7
S$17359
  Bottom 0: 85.19,87.7 85.5,87.8
S$17360
  Bottom 0: 85.5,87.8 85.78,87.97
S$17361
  Bottom 0: 85.78,87.97 85.99,88.22
S$17362
  Bottom 0: 85.99,88.22 86.13,88.52
S$17363
  Bottom 0: 86.13,88.52 86.17,88.84
S$17364
  Bottom 0: 86.17,88.84 86.13,89.16
S$17365
  Bottom 0: 86.13,89.16 85.99,89.46
S$17366
  Bottom 0: 85.99,89.46 85.82,89.65
S$17367
  Bottom 0: 85.82,89.65 100.39,89.65
S$17368
  Bottom 0: 100.39,89.65 100.39,87.95
S$17369
  Bottom 0: 100.39,87.95 100.4,87.87
S$17370
  Bottom 0: 100.4,87.87 100.44,87.8
S$17371
  Bottom 0: 100.44,87.8 100.5,87.74
S$17372
  Bottom 0: 100.5,87.74 100.57,87.7
S$17373
  Bottom 0: 100.57,87.7 100.65,87.69
S$17374
  Bottom 0: 100.65,87.69 101.04,87.69
S$17375
  Bottom 0: 101.04,87.69 98.2,84.86
S$17376
  Bottom 0: 98.2,84.86 98.15,84.8
S$17377
  Bottom 0: 98.15,84.8 98.12,84.75
S$17378
  Bottom 0: 98.12,84.75 98.08,84.68
S$17379
  Bottom 0: 98.08,84.68 98.07,84.61
S$17380
  Bottom 0: 98.07,84.61 98.07,84.54
S$17381
  Bottom 0: 98.07,84.54 98.07,76.14
S$17382
  Bottom 0: 98.07,76.14 97.91,75.89
S$17383
  Bottom 0: 97.91,75.89 97.82,75.58
S$17384
  Bottom 0: 97.82,75.58 97.82,75.25
S$17385
  Bottom 0: 97.82,75.25 97.91,74.94
S$17386
  Bottom 0: 97.91,74.94 97.99,74.81
S$17387
  Bottom 0: 97.99,74.81 95.75,77.05
S$17388
  Bottom 0: 95.75,77.05 95.7,77.09
S$17389
  Bottom 0: 95.7,77.09 95.64,77.13
S$17390
  Bottom 0: 95.64,77.13 95.58,77.15
S$17391
  Bottom 0: 95.58,77.15 95.51,77.17
S$17392
  Bottom 0: 95.51,77.17 95.44,77.17
S$17393
  Bottom 0: 95.44,77.17 92.23,77.17
S$17394
  Bottom 0: 92.23,77.17 88.81,80.6
S$17395
  Bottom 0: 88.81,80.6 88.92,80.87
S$17396
  Bottom 0: 88.92,80.87 88.97,81.22
S$17397
  Bottom 0: 88.97,81.22 88.92,81.56
S$17398
  Bottom 0: 88.92,81.56 88.8,81.89
S$17399
  Bottom 0: 88.8,81.89 88.59,82.17
S$17400
  Bottom 0: 88.59,82.17 88.32,82.39
S$17401
  Bottom 0: 88.32,82.39 88,82.55
S$17402
  Bottom 0: 88,82.55 87.66,82.61
S$17403
  Bottom 0: 87.66,82.61 87.31,82.59
S$17404
  Bottom 0: 87.31,82.59 86.97,82.48
S$17405
  Bottom 0: 86.97,82.48 86.68,82.29
S$17406
  Bottom 0: 86.68,82.29 86.44,82.04
S$17407
  Bottom 0: 86.44,82.04 86.27,81.73
S$17408
  Bottom 0: 86.27,81.73 86.18,81.39
S$17409
  Bottom 0: 86.18,81.39 86.18,81.04
S$17410
  Bottom 0: 86.18,81.04 86.27,80.7
S$17411
  Bottom 0: 86.27,80.7 86.44,80.39
S$17412
  Bottom 0: 86.44,80.39 86.68,80.14
S$17413
  Bottom 0: 86.68,80.14 86.97,79.95
S$17414
  Bottom 0: 86.97,79.95 87.31,79.84
S$17415
  Bottom 0: 87.31,79.84 87.66,79.83
S$17416
  Bottom 0: 87.66,79.83 88,79.89
S$17417
  Bottom 0: 88,79.89 88.19,79.98
S$17418
  Bottom 0: 88.19,79.98 91.73,76.42
S$17419
  Bottom 0: 91.73,76.42 91.79,76.38
S$17420
  Bottom 0: 91.79,76.38 91.85,76.33
S$17421
  Bottom 0: 91.85,76.33 91.92,76.31
S$17422
  Bottom 0: 91.92,76.31 91.98,76.29
S$17423
  Bottom 0: 91.98,76.29 92.05,76.29
S$17424
  Bottom 0: 92.05,76.29 95.25,76.29
S$17425
  Bottom 0: 95.25,76.29 97.33,74.21
S$17426
  Bottom 0: 97.33,74.21 97.02,74.23
S$17427
  Bottom 0: 97.02,74.23 96.77,74.18
S$17428
  Bottom 0: 96.77,74.18 95.13,75.82
S$17429
  Bottom 0: 95.13,75.82 95.06,75.88
S$17430
  Bottom 0: 95.06,75.88 94.98,75.93
S$17431
  Bottom 0: 94.98,75.93 94.9,75.96
S$17432
  Bottom 0: 94.9,75.96 94.82,75.98
S$17433
  Bottom 0: 94.82,75.98 94.72,75.99
S$17434
  Bottom 0: 94.72,75.99 88.62,75.99
S$17435
  Bottom 0: 88.62,75.99 88.59,76.04
S$17436
  Bottom 0: 88.59,76.04 88.39,76.29
S$17437
  Bottom 0: 88.39,76.29 88.12,76.48
S$17438
  Bottom 0: 88.12,76.48 87.82,76.59
S$17439
  Bottom 0: 87.82,76.59 87.5,76.61
S$17440
  Bottom 0: 87.5,76.61 87.17,76.54
S$17441
  Bottom 0: 87.17,76.54 86.89,76.4
S$17442
  Bottom 0: 86.89,76.4 86.65,76.17
S$17443
  Bottom 0: 86.65,76.17 86.48,75.89
S$17444
  Bottom 0: 86.48,75.89 86.39,75.58
S$17445
  Bottom 0: 86.39,75.58 86.39,75.26
S$17446
  Bottom 0: 86.39,75.26 86.44,75.08
S$17447
  Bottom 0: 86.44,75.08 84.97,73.61
S$17448
  Bottom 0: 84.97,73.61 79.09,73.61
S$17449
  Bottom 0: 93.37,79.17 93.66,79.23
S$17450
  Bottom 0: 93.66,79.23 93.93,79.39
S$17451
  Bottom 0: 93.93,79.39 94.13,79.61
S$17452
  Bottom 0: 94.13,79.61 94.26,79.88
S$17453
  Bottom 0: 94.26,79.88 94.31,80.18
S$17454
  Bottom 0: 94.31,80.18 94.26,80.48
S$17455
  Bottom 0: 94.26,80.48 94.13,80.75
S$17456
  Bottom 0: 94.13,80.75 93.93,80.97
S$17457
  Bottom 0: 93.93,80.97 93.66,81.12
S$17458
  Bottom 0: 93.66,81.12 93.37,81.19
S$17459
  Bottom 0: 93.37,81.19 93.06,81.17
S$17460
  Bottom 0: 93.06,81.17 92.78,81.06
S$17461
  Bottom 0: 92.78,81.06 92.55,80.87
S$17462
  Bottom 0: 92.55,80.87 92.38,80.62
S$17463
  Bottom 0: 92.38,80.62 92.29,80.33
S$17464
  Bottom 0: 92.29,80.33 92.29,80.03
S$17465
  Bottom 0: 92.29,80.03 92.38,79.74
S$17466
  Bottom 0: 92.38,79.74 92.55,79.49
S$17467
  Bottom 0: 92.55,79.49 92.78,79.3
S$17468
  Bottom 0: 92.78,79.3 93.06,79.19
S$17469
  Bottom 0: 93.06,79.19 93.37,79.17
S$17470
  Bottom 0: 75.51,79.17 75.8,79.24
S$17471
  Bottom 0: 75.8,79.24 76.06,79.39
S$17472
  Bottom 0: 76.06,79.39 76.27,79.61
S$17473
  Bottom 0: 76.27,79.61 76.4,79.89
S$17474
  Bottom 0: 76.4,79.89 76.45,80.19
S$17475
  Bottom 0: 76.45,80.19 76.4,80.48
S$17476
  Bottom 0: 76.4,80.48 76.27,80.76
S$17477
  Bottom 0: 76.27,80.76 76.06,80.98
S$17478
  Bottom 0: 76.06,80.98 75.8,81.13
S$17479
  Bottom 0: 75.8,81.13 75.51,81.2
S$17480
  Bottom 0: 75.51,81.2 75.2,81.18
S$17481
  Bottom 0: 75.2,81.18 74.92,81.06
S$17482
  Bottom 0: 74.92,81.06 74.68,80.88
S$17483
  Bottom 0: 74.68,80.88 74.52,80.63
S$17484
  Bottom 0: 74.52,80.63 74.42,80.34
S$17485
  Bottom 0: 74.42,80.34 74.42,80.03
S$17486
  Bottom 0: 74.42,80.03 74.52,79.74
S$17487
  Bottom 0: 74.52,79.74 74.68,79.49
S$17488
  Bottom 0: 74.68,79.49 74.92,79.31
S$17489
  Bottom 0: 74.92,79.31 75.2,79.19
S$17490
  Bottom 0: 75.2,79.19 75.51,79.17
S$17491
  Bottom 0: 83.76,81.47 84.21,81.52
S$17492
  Bottom 0: 84.21,81.52 84.64,81.64
S$17493
  Bottom 0: 84.64,81.64 85.03,81.86
S$17494
  Bottom 0: 85.03,81.86 85.38,82.14
S$17495
  Bottom 0: 85.38,82.14 85.66,82.49
S$17496
  Bottom 0: 85.66,82.49 85.88,82.88
S$17497
  Bottom 0: 85.88,82.88 86,83.31
S$17498
  Bottom 0: 86,83.31 86.05,83.76
S$17499
  Bottom 0: 86.05,83.76 86,84.2
S$17500
  Bottom 0: 86,84.2 85.88,84.63
S$17501
  Bottom 0: 85.88,84.63 85.66,85.03
S$17502
  Bottom 0: 85.66,85.03 85.38,85.37
S$17503
  Bottom 0: 85.38,85.37 85.03,85.66
S$17504
  Bottom 0: 85.03,85.66 84.64,85.87
S$17505
  Bottom 0: 84.64,85.87 84.21,86
S$17506
  Bottom 0: 84.21,86 83.76,86.04
S$17507
  Bottom 0: 83.76,86.04 83.31,86
S$17508
  Bottom 0: 83.31,86 82.89,85.87
S$17509
  Bottom 0: 82.89,85.87 82.49,85.66
S$17510
  Bottom 0: 82.49,85.66 82.14,85.37
S$17511
  Bottom 0: 82.14,85.37 81.86,85.03
S$17512
  Bottom 0: 81.86,85.03 81.65,84.63
S$17513
  Bottom 0: 81.65,84.63 81.52,84.2
S$17514
  Bottom 0: 81.52,84.2 81.48,83.76
S$17515
  Bottom 0: 81.48,83.76 81.52,83.31
S$17516
  Bottom 0: 81.52,83.31 81.65,82.88
S$17517
  Bottom 0: 81.65,82.88 81.86,82.49
S$17518
  Bottom 0: 81.86,82.49 82.14,82.14
S$17519
  Bottom 0: 82.14,82.14 82.49,81.86
S$17520
  Bottom 0: 82.49,81.86 82.89,81.64
S$17521
  Bottom 0: 82.89,81.64 83.31,81.52
S$17522
  Bottom 0: 83.31,81.52 83.76,81.47
S$17523
  Bottom 0: 93.37,86.79 93.66,86.86
S$17524
  Bottom 0: 93.66,86.86 93.93,87.01
S$17525
  Bottom 0: 93.93,87.01 94.13,87.23
S$17526
  Bottom 0: 94.13,87.23 94.26,87.5
S$17527
  Bottom 0: 94.26,87.5 94.31,87.8
S$17528
  Bottom 0: 94.31,87.8 94.26,88.1
S$17529
  Bottom 0: 94.26,88.1 94.13,88.37
S$17530
  Bottom 0: 94.13,88.37 93.93,88.59
S$17531
  Bottom 0: 93.93,88.59 93.66,88.75
S$17532
  Bottom 0: 93.66,88.75 93.37,88.81
S$17533
  Bottom 0: 93.37,88.81 93.06,88.79
S$17534
  Bottom 0: 93.06,88.79 92.78,88.68
S$17535
  Bottom 0: 92.78,88.68 92.55,88.49
S$17536
  Bottom 0: 92.55,88.49 92.38,88.24
S$17537
  Bottom 0: 92.38,88.24 92.29,87.95
S$17538
  Bottom 0: 92.29,87.95 92.29,87.65
S$17539
  Bottom 0: 92.29,87.65 92.38,87.36
S$17540
  Bottom 0: 92.38,87.36 92.55,87.11
S$17541
  Bottom 0: 92.55,87.11 92.78,86.92
S$17542
  Bottom 0: 92.78,86.92 93.06,86.81
S$17543
  Bottom 0: 93.06,86.81 93.37,86.79
S$17544
  Bottom 0: 137.76,74.42 137.93,74.54
S$17545
  Bottom 0: 137.93,74.54 138.13,74.8
S$17546
  Bottom 0: 138.13,74.8 138.26,75.09
S$17547
  Bottom 0: 138.26,75.09 138.31,75.42
S$17548
  Bottom 0: 138.31,75.42 138.26,75.73
S$17549
  Bottom 0: 138.26,75.73 138.13,76.03
S$17550
  Bottom 0: 138.13,76.03 137.93,76.29
S$17551
  Bottom 0: 137.93,76.29 137.66,76.48
S$17552
  Bottom 0: 137.66,76.48 137.36,76.58
S$17553
  Bottom 0: 137.36,76.58 137.12,76.6
S$17554
  Bottom 0: 137.12,76.6 137.12,78.06
S$17555
  Bottom 0: 137.12,78.06 137.24,77.85
S$17556
  Bottom 0: 137.24,77.85 137.48,77.6
S$17557
  Bottom 0: 137.48,77.6 137.77,77.41
S$17558
  Bottom 0: 137.77,77.41 138.1,77.31
S$17559
  Bottom 0: 138.1,77.31 138.45,77.28
S$17560
  Bottom 0: 138.45,77.28 138.8,77.35
S$17561
  Bottom 0: 138.8,77.35 139.11,77.5
S$17562
  Bottom 0: 139.11,77.5 139.38,77.72
S$17563
  Bottom 0: 139.38,77.72 139.59,78.01
S$17564
  Bottom 0: 139.59,78.01 139.72,78.33
S$17565
  Bottom 0: 139.72,78.33 139.76,78.68
S$17566
  Bottom 0: 139.76,78.68 139.72,79.02
S$17567
  Bottom 0: 139.72,79.02 139.61,79.3
S$17568
  Bottom 0: 139.61,79.3 142.49,76.42
S$17569
  Bottom 0: 142.49,76.42 142.54,76.37
S$17570
  Bottom 0: 142.54,76.37 142.6,76.33
S$17571
  Bottom 0: 142.6,76.33 142.66,76.3
S$17572
  Bottom 0: 142.66,76.3 142.73,76.29
S$17573
  Bottom 0: 142.73,76.29 142.8,76.28
S$17574
  Bottom 0: 142.8,76.28 143.93,76.28
S$17575
  Bottom 0: 143.93,76.28 143.81,76.17
S$17576
  Bottom 0: 143.81,76.17 143.63,75.89
S$17577
  Bottom 0: 143.63,75.89 143.55,75.58
S$17578
  Bottom 0: 143.55,75.58 143.55,75.25
S$17579
  Bottom 0: 143.55,75.25 143.63,74.94
S$17580
  Bottom 0: 143.63,74.94 143.81,74.66
S$17581
  Bottom 0: 143.81,74.66 144.04,74.44
S$17582
  Bottom 0: 144.04,74.44 144.07,74.42
S$17583
  Bottom 0: 144.07,74.42 137.76,74.42
S$17584
  Bottom 0: 118.87,74.55 119.08,74.8
S$17585
  Bottom 0: 119.08,74.8 119.2,75.1
S$17586
  Bottom 0: 119.2,75.1 119.25,75.42
S$17587
  Bottom 0: 119.25,75.42 119.2,75.74
S$17588
  Bottom 0: 119.2,75.74 119.08,76.04
S$17589
  Bottom 0: 119.08,76.04 118.87,76.29
S$17590
  Bottom 0: 118.87,76.29 118.61,76.48
S$17591
  Bottom 0: 118.61,76.48 118.3,76.59
S$17592
  Bottom 0: 118.3,76.59 118.18,76.59
S$17593
  Bottom 0: 118.18,76.59 118.18,77.86
S$17594
  Bottom 0: 118.18,77.86 118.19,77.85
S$17595
  Bottom 0: 118.19,77.85 118.43,77.6
S$17596
  Bottom 0: 118.43,77.6 118.72,77.41
S$17597
  Bottom 0: 118.72,77.41 119.05,77.31
S$17598
  Bottom 0: 119.05,77.31 119.4,77.28
S$17599
  Bottom 0: 119.4,77.28 119.75,77.35
S$17600
  Bottom 0: 119.75,77.35 120.06,77.5
S$17601
  Bottom 0: 120.06,77.5 120.33,77.72
S$17602
  Bottom 0: 120.33,77.72 120.54,78.01
S$17603
  Bottom 0: 120.54,78.01 120.67,78.33
S$17604
  Bottom 0: 120.67,78.33 120.71,78.68
S$17605
  Bottom 0: 120.71,78.68 120.67,79.02
S$17606
  Bottom 0: 120.67,79.02 120.54,79.35
S$17607
  Bottom 0: 120.54,79.35 120.33,79.63
S$17608
  Bottom 0: 120.33,79.63 120.06,79.86
S$17609
  Bottom 0: 120.06,79.86 119.75,80.01
S$17610
  Bottom 0: 119.75,80.01 119.4,80.07
S$17611
  Bottom 0: 119.4,80.07 119.05,80.05
S$17612
  Bottom 0: 119.05,80.05 118.72,79.94
S$17613
  Bottom 0: 118.72,79.94 118.43,79.75
S$17614
  Bottom 0: 118.43,79.75 118.19,79.5
S$17615
  Bottom 0: 118.19,79.5 118.18,79.49
S$17616
  Bottom 0: 118.18,79.49 118.18,84.54
S$17617
  Bottom 0: 118.18,84.54 120.9,87.25
S$17618
  Bottom 0: 120.9,87.25 120.93,87.31
S$17619
  Bottom 0: 120.93,87.31 120.97,87.35
S$17620
  Bottom 0: 120.97,87.35 120.98,87.39
S$17621
  Bottom 0: 120.98,87.39 121.01,87.45
S$17622
  Bottom 0: 121.01,87.45 121.01,87.51
S$17623
  Bottom 0: 121.01,87.51 121.03,87.57
S$17624
  Bottom 0: 121.03,87.57 121.03,87.69
S$17625
  Bottom 0: 121.03,87.69 121.47,87.69
S$17626
  Bottom 0: 121.47,87.69 121.55,87.7
S$17627
  Bottom 0: 121.55,87.7 121.62,87.74
S$17628
  Bottom 0: 121.62,87.74 121.68,87.8
S$17629
  Bottom 0: 121.68,87.8 121.72,87.87
S$17630
  Bottom 0: 121.72,87.87 121.73,87.95
S$17631
  Bottom 0: 121.73,87.95 121.73,89.65
S$17632
  Bottom 0: 121.73,89.65 122.34,89.65
S$17633
  Bottom 0: 122.34,89.65 122.17,89.46
S$17634
  Bottom 0: 122.17,89.46 122.03,89.16
S$17635
  Bottom 0: 122.03,89.16 121.98,88.84
S$17636
  Bottom 0: 121.98,88.84 122.03,88.52
S$17637
  Bottom 0: 122.03,88.52 122.17,88.22
S$17638
  Bottom 0: 122.17,88.22 122.38,87.97
S$17639
  Bottom 0: 122.38,87.97 122.65,87.8
S$17640
  Bottom 0: 122.65,87.8 122.96,87.7
S$17641
  Bottom 0: 122.96,87.7 123.29,87.7
S$17642
  Bottom 0: 123.29,87.7 123.6,87.8
S$17643
  Bottom 0: 123.6,87.8 123.87,87.97
S$17644
  Bottom 0: 123.87,87.97 124.09,88.22
S$17645
  Bottom 0: 124.09,88.22 124.22,88.52
S$17646
  Bottom 0: 124.22,88.52 124.27,88.84
S$17647
  Bottom 0: 124.27,88.84 124.22,89.16
S$17648
  Bottom 0: 124.22,89.16 124.09,89.46
S$17649
  Bottom 0: 124.09,89.46 123.91,89.65
S$17650
  Bottom 0: 123.91,89.65 138.49,89.65
S$17651
  Bottom 0: 138.49,89.65 138.49,87.95
S$17652
  Bottom 0: 138.49,87.95 138.5,87.87
S$17653
  Bottom 0: 138.5,87.87 138.54,87.8
S$17654
  Bottom 0: 138.54,87.8 138.6,87.74
S$17655
  Bottom 0: 138.6,87.74 138.67,87.7
S$17656
  Bottom 0: 138.67,87.7 138.75,87.69
S$17657
  Bottom 0: 138.75,87.69 139.14,87.69
S$17658
  Bottom 0: 139.14,87.69 136.37,84.93
S$17659
  Bottom 0: 136.37,84.93 136.32,84.87
S$17660
  Bottom 0: 136.32,84.87 136.29,84.82
S$17661
  Bottom 0: 136.29,84.82 136.26,84.75
S$17662
  Bottom 0: 136.26,84.75 136.24,84.69
S$17663
  Bottom 0: 136.24,84.69 136.24,84.61
S$17664
  Bottom 0: 136.24,84.61 136.24,76.22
